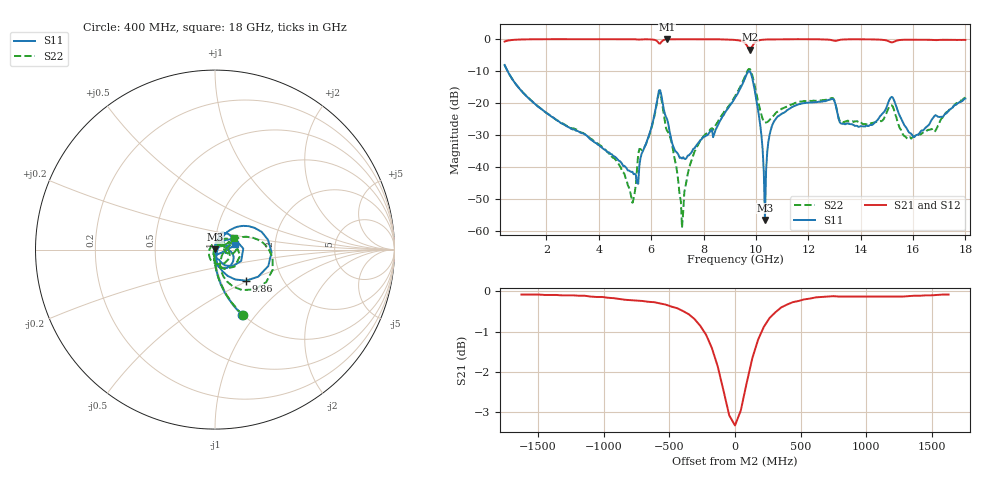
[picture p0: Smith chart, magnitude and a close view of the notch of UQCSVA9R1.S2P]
!  Part Number  UQCSVA9R1  Mounting Orientation: Horizontal
!  Description: Ultra Low ESR Microwave capacitors
!  Application: Coupling, Bypass, Tuning, DC Block
!  Filters, Matching
# GHZ S DB R 50
! Freq  |S11|  S11 Ph  |S21|  S21 Ph  |S12|  S12 Ph  |S22|  S22 Ph
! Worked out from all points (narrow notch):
!   401 points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, 400 MHz to 18 GHz, reference 50 ohm
!   highest |S21| = -0.03 dB at 6.604 GHz (marker M1); lowest = -3.3 dB at 9.772 GHz (marker M2)
!   notch at M2: 3.2 dB deep, 273 MHz wide at half that depth
!   lowest |S11| = -56.5 dB at 10.34 GHz (marker M3), VSWR 1.00, Z = 49.9 + j0.0709 ohm
!   |S11| at or under -10 dB: 511.3 MHz to end of sweep
!   |S22| runs from -58.9 to -8.1 dB; largest |S21 - S12| = 0.0086
!   S11 on the Smith chart (normalised r, x): 400 MHz: 0.99, -0.85; 9.86 GHz: 1.32, -0.48; 18 GHz: 1.25, +0.09
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0.4  -8.12 -67.3  -0.80 22.1  -0.80 22.1  -8.07 -66.9
3.348  -29.42 -92.9  -0.06 -9.5  -0.06 -9.4  -29.26 -94.6
4.668  -37.13 -78.6  -0.05 -15.5  -0.05 -15.4  -38.10 -103.3
5.284  -41.45 -42.6  -0.07 -18.5  -0.07 -18.5  -51.14 -148.5
5.504  -45.21 179.5  -0.19 -19.5  -0.19 -19.4  -35.89 121.0
6.296  -16.05 2.1  -1.38 -24.1  -1.36 -23.9  -16.79 -13.4
6.604  -24.95 -72.5  -0.03 -20.6  -0.03 -20.4  -28.70 -92.2
7.176  -37.30 -25.5  -0.08 -24.7  -0.07 -24.5  -58.90 155.3
7.748  -32.96 30.0  -0.07 -27.5  -0.07 -27.4  -33.61 59.5
9.2  -18.35 55.4  -0.30 -36.6  -0.29 -36.5  -17.89 28.4
9.772  -10.15 -17.1  -3.33 -32.8  -3.30 -32.7  -9.42 -32.4
9.86  -12.24 -45.1  -2.29 -23.8  -2.27 -23.8  -11.30 -56.0
10.344  -56.47 151.7  -0.18 -31.7  -0.17 -31.6  -26.16 -34.5
10.52  -29.96 86.1  -0.12 -33.7  -0.12 -33.6  -25.30 -6.9
10.74  -25.15 75.4  -0.13 -35.4  -0.13 -35.3  -23.32 7.8
12.148  -19.81 66.0  -0.08 -43.3  -0.08 -43.2  -19.35 20.4
12.896  -18.73 44.6  -0.37 -47.7  -0.36 -47.6  -18.43 6.4
13.248  -26.40 34.4  -0.22 -46.0  -0.21 -45.8  -25.98 2.8
13.996  -27.22 45.2  -0.10 -50.6  -0.08 -50.5  -25.93 25.1
15.096  -19.00 -21.9  -0.81 -57.4  -0.79 -57.1  -21.07 -21.6
16.064  -30.54 -54.9  -0.22 -57.7  -0.21 -57.4  -30.24 122.0
18  -18.60 16.7  -0.29 -66.0  -0.28 -65.8  -18.30 31.9
